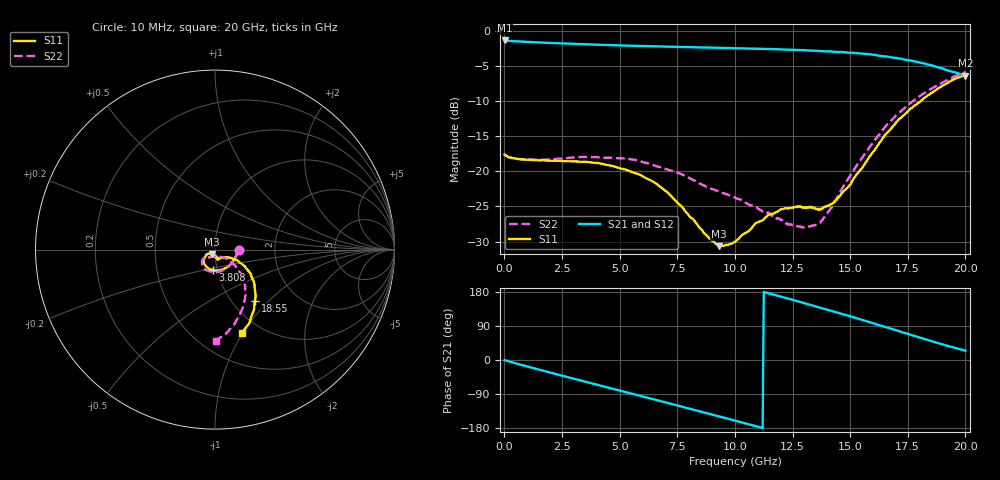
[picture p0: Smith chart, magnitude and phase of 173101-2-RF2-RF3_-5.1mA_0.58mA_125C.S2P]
!  2-Port S-parameters saved by WinCal
! VAR MeasName=S-Parameters (CALIBRATED_DATA) read from VNA (N5242A)
! VAR MeasDate=2017-7-20 10:55:46
! VAR NAME=173101-2-RF2-RF3_-5.1mA_0.58mA_125C
! VAR FILENAME=173101-2-RF2-RF3_-5.1mA_0.58mA_125C.S2P
! VAR DATE=2017-7-20 10:55:47
! VAR PHYS_PORTS=1,2
# Hz S DB R 50
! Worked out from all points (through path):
!   401 points, 10 MHz to 20 GHz, reference 50 ohm
!   highest |S21| = -1.40 dB at 10 MHz (marker M1); lowest = -6.4 dB at 20 GHz (marker M2)
!   group delay of S21, straight-line fit = 46.2 ps
!   lowest |S11| = -30.6 dB at 9.305 GHz (marker M3), VSWR 1.06, Z = 48.4 - j2.44 ohm
!   |S11| at or under -10 dB: start of sweep to 18.06 GHz
!   |S22| runs from -28.0 to -5.9 dB; largest |S21 - S12| = 0.0061
!   S11 on the Smith chart (normalised r, x): 10 MHz: 1.30, -0.01; 3.808 GHz: 0.95, -0.22; 18.55 GHz: 1.27, -0.83; 20 GHz: 0.82, -0.99
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1e7  -17.62 -1.0  -1.40 -0.2  -1.40 -0.2  -17.61 -1.0
8.096e8  -18.31 -25.2  -1.57 -14.0  -1.57 -14.1  -18.28 -25.5
1.559225e9  -18.45 -45.6  -1.69 -26.3  -1.69 -26.3  -18.38 -45.9
2.50875e9  -18.54 -69.1  -1.82 -41.5  -1.83 -41.5  -18.20 -68.7
3.358325e9  -18.64 -87.9  -1.93 -54.9  -1.94 -54.9  -17.95 -85.9
3.8081e9  -18.76 -96.2  -1.98 -62.0  -1.98 -62.0  -17.99 -93.6
5.2074e9  -19.71 -121.8  -2.13 -83.9  -2.14 -83.8  -18.15 -115.7
6.70665e9  -22.06 -139.3  -2.24 -107.4  -2.24 -107.3  -19.37 -131.5
7.956025e9  -26.09 -149.3  -2.33 -127.0  -2.35 -127.1  -20.84 -140.9
9.30535e9  -30.64 -121.1  -2.44 -148.6  -2.44 -148.7  -22.87 -140.5
1.0005e10  -29.99 -92.7  -2.50 -159.9  -2.51 -160.0  -23.74 -137.0
1.090455e10  -27.35 -78.3  -2.57 -174.5  -2.58 -174.6  -25.09 -128.1
1.165418e10  -26.04 -78.1  -2.63 173.0  -2.64 173.0  -26.38 -122.9
1.24038e10  -25.21 -76.4  -2.72 160.4  -2.72 160.4  -27.58 -113.1
1.335332e10  -25.07 -69.6  -2.85 144.3  -2.83 144.3  -27.72 -84.1
1.375312e10  -25.30 -61.1  -2.91 137.3  -2.91 137.3  -27.00 -65.5
1.44028e10  -24.10 -44.2  -3.03 126.0  -3.05 126.0  -23.90 -43.6
1.555222e10  -19.38 -26.9  -3.28 105.2  -3.30 105.1  -17.94 -38.1
1.670165e10  -14.17 -29.8  -3.74 83.8  -3.80 83.6  -13.04 -45.7
1.76012e10  -11.16 -39.0  -4.25 67.3  -4.25 67.2  -10.32 -56.2
1.855072e10  -8.83 -52.1  -4.95 49.3  -5.02 49.5  -8.20 -69.3
2e10  -6.25 -72.0  -6.40 24.6  -6.46 25.1  -5.91 -89.6
